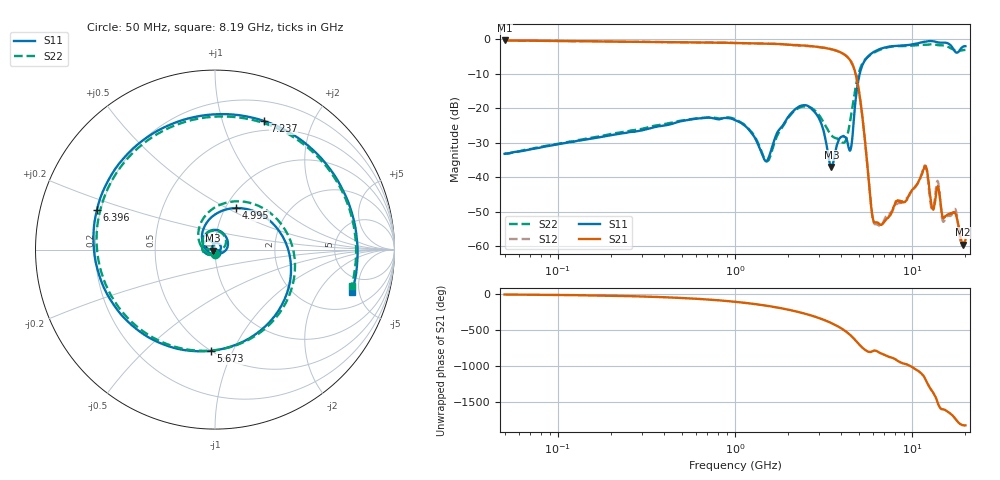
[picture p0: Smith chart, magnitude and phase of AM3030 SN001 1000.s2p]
# Hz S DB R 50
!freq MagS11 AngS11 MagS21 AngS21 MagS12 AngS12 MagS22 AngS22
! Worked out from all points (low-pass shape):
!   1601 points, 50 MHz to 20.05 GHz, reference 50 ohm
!   highest |S21| = -0.41 dB at 50 MHz (marker M1); lowest = -59.5 dB at 19.39 GHz (marker M2)
!   |S21| within 3 dB of the highest: start of sweep to 3.764 GHz
!   lowest |S11| = -37.0 dB at 3.512 GHz (marker M3), VSWR 1.03, Z = 48.8 - j0.651 ohm
!   |S11| at or under -10 dB: start of sweep to 5.075 GHz
!   |S22| runs from -35.4 to -1.5 dB; largest |S21 - S12| = 0.012
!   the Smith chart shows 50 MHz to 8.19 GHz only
!   S11 on the Smith chart (normalised r, x): 50 MHz: 1.00, -0.04; 4.995 GHz: 1.12, +0.56; 5.673 GHz: 0.50, -0.83; 6.396 GHz: 0.19, +0.16; 7.237 GHz: 0.40, +1.38; 8.19 GHz: 3.20, -4.21
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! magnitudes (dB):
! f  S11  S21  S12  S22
! 50 MHz  -33.2  -0.4  -0.4  -33.1
! 135.9 MHz  -29.3  -0.6  -0.6  -29.1
! 369.6 MHz  -25.3  -0.9  -0.9  -24.9
! 1.005 GHz  -23.5  -1.2  -1.1  -23.2
! 1.523 GHz  -35.1  -1.4  -1.4  -35.4
! 2.071 GHz  -21.6  -1.7  -1.7  -21.8
! 2.722 GHz  -20.3  -2.1  -2.1  -20.0
! 3.512 GHz  -37.0  -3.0  -3.0  -27.9
! 4.497 GHz  -32.1  -6.3  -6.3  -23.2
! 4.995 GHz  -11.7  -14.3  -14.3  -10.1
! 5.673 GHz  -5.0  -39.7  -39.6  -5.1
! 6.396 GHz  -3.2  -53.1  -53.7  -3.4
! 7.237 GHz  -2.3  -51.9  -51.0  -2.4
! 7.402 GHz  -2.2  -51.4  -50.7  -2.3
! 8.19 GHz  -1.9  -47.0  -47.8  -2.1
! 11.82 GHz  -0.8  -36.8  -36.6  -1.7
! 12.93 GHz  -0.6  -48.6  -49.1  -1.5
! 13.99 GHz  -1.0  -42.6  -41.1  -1.8
! 15.03 GHz  -1.0  -51.8  -52.9  -1.9
! 17.52 GHz  -3.6  -50.4  -49.2  -3.3
! 19.39 GHz  -2.3  -59.5  -59.7  -3.2
! 20.05 GHz  -2.1  -58.2  -58.6  -3.2
